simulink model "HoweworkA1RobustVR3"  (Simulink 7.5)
settings: Solver=ode45  StartTime=0.0  StopTime=10.0  RelTol=1e-3

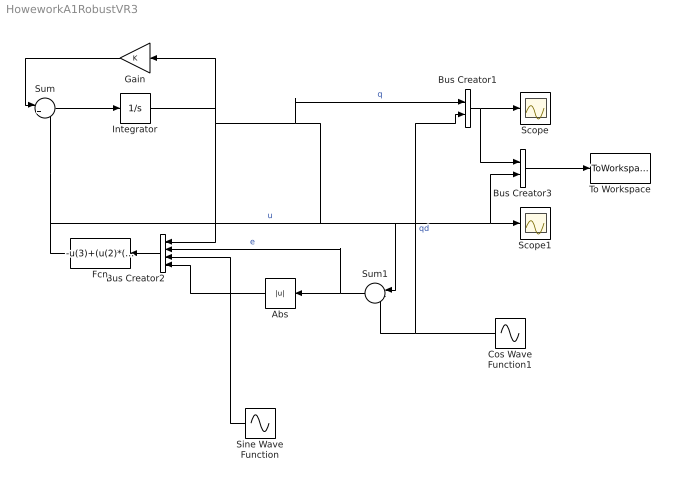
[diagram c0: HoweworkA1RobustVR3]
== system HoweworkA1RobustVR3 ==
  Abs : Abs  OutDataType=fixdt(1, 16)  OutScaling=2^0
  Bus Creator1 : BusCreator  Inputs=2
  Bus Creator2 : BusCreator
  Bus Creator3 : BusCreator  Inputs=2
  Cos Wave Function1 : Sin  Amplitude=1  Bias=0  Frequency=1  Phase=pi/2  Samples=10  SampleTime=0
  Fcn : Fcn  Expr=-u(3)+(u(2)*(u(1)*u(1)+1)^2)/((u(1)*u(1)+1)*u(4)+.5)+1*(u(2))
  Gain : Gain  ParameterDataType=fixdt(1, 16)  ParameterScaling=2^0  OutDataType=fixdt(1, 16)  OutScaling=2^0
  Integrator : Integrator
  Scope : Scope
  Scope1 : Scope
  Sine Wave Function : Sin  Amplitude=1  Bias=0  Frequency=1  Phase=0  Samples=10  SampleTime=0
  Sum : Sum  Inputs=|++  OutDataType=fixdt(1, 16)  OutScaling=2^0
  Sum1 : Sum  Inputs=|-+  OutDataType=fixdt(1, 16)  OutScaling=2^0
  To Workspace : ToWorkspace  VariableName=ICP  SampleTime=-1  SaveFormat=Structure With Time
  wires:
  Integrator/1 -> Gain/1, Bus Creator2/1, Bus Creator1/1, Sum1/1  "q"
  Sum/1 -> Integrator/1
  Gain/1 -> Sum/1
  Bus Creator1/1 -> Scope/1, Bus Creator3/1
  Fcn/1 -> Sum/2, Scope1/1, Bus Creator3/2  "u"
  Bus Creator2/1 -> Fcn/1
  Cos Wave Function1/1 -> Sum1/2, Bus Creator1/2  "qd"
  Sum1/1 -> Bus Creator2/2, Abs/1  "e"
  Sine Wave Function/1 -> Bus Creator2/3
  Abs/1 -> Bus Creator2/4
  Bus Creator3/1 -> To Workspace/1
